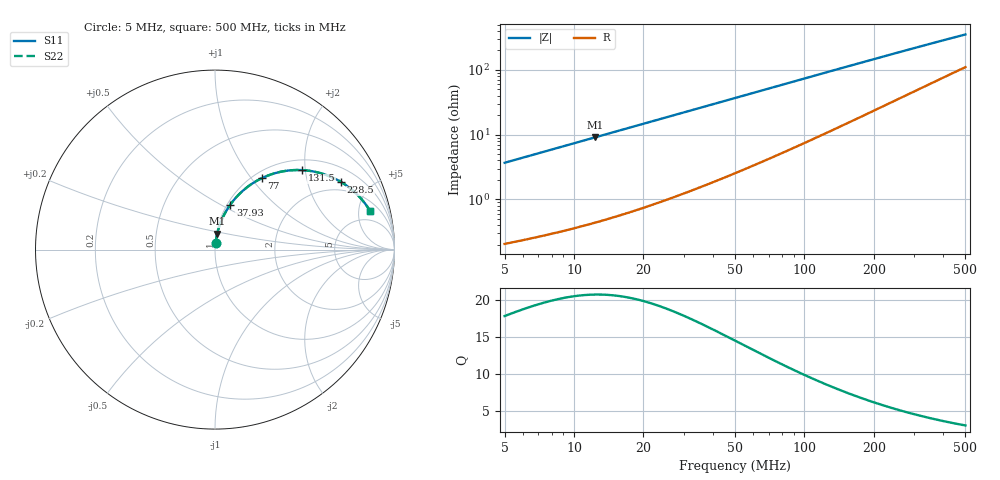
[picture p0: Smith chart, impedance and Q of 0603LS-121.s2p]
# MHz S MA R 50
!Freq  MagS11  AngS11  MagS21  AngS21  MagS12  AngS12  MagS22  AngS22
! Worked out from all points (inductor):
!   801 points, 5 MHz to 500 MHz, reference 50 ohm
!   read as one part in series: L = 117 nH near 5.116 MHz
!   highest Q = 20.7 at 12.34 MHz (marker M1), where L = 117 nH
!   S11 on the Smith chart (normalised r, x): 5 MHz: 1.00, +0.07; 37.93 MHz: 1.03, +0.56; 77 MHz: 1.10, +1.13; 131.5 MHz: 1.23, +1.92; 228.5 MHz: 1.59, +3.27; 500 MHz: 3.20, +6.67
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5  0.0367 84.7  0.9973 -2.1  0.9973 -2.1  0.0367 84.7
6.55345  0.04806 84.3  0.9963 -2.8  0.9963 -2.8  0.04806 84.3
8.202949  0.06011 83.7  0.9952 -3.4  0.9952 -3.4  0.06011 83.7
10.15009  0.07428 83.0  0.9936 -4.3  0.9936 -4.3  0.07428 83.0
12.3444  0.09019 82.1  0.9916 -5.2  0.9916 -5.2  0.09019 82.1
17.04002  0.1239 80.1  0.9862 -7.1  0.9862 -7.1  0.1239 80.1
22.85441  0.1648 77.6  0.9778 -9.5  0.9778 -9.5  0.1648 77.6
29.78311  0.2121 74.6  0.9655 -12.2  0.9655 -12.2  0.2121 74.6
37.92888  0.2653 71.2  0.9482 -15.4  0.9482 -15.4  0.2653 71.2
46.12857  0.3157 67.8  0.9282 -18.4  0.9282 -18.4  0.3157 67.8
55.14041  0.3674 64.4  0.9039 -21.5  0.9039 -21.5  0.3674 64.4
76.99633  0.4759 56.7  0.8394 -28.3  0.8394 -28.3  0.4759 56.7
87.89618  0.5214 53.4  0.8061 -31.3  0.8061 -31.3  0.5214 53.4
108.1359  0.5924 47.8  0.7453 -36.1  0.7453 -36.1  0.5924 47.8
131.5134  0.6562 42.5  0.6799 -40.6  0.6799 -40.6  0.6562 42.5
170.4002  0.7307 35.5  0.5861 -46.3  0.5861 -46.3  0.7307 35.5
197.911  0.7671 31.6  0.5311 -49.2  0.5311 -49.2  0.7671 31.6
228.5441  0.7972 28.2  0.4794 -51.7  0.4794 -51.7  0.7972 28.2
253.4954  0.816 25.8  0.4435 -53.2  0.4435 -53.2  0.816 25.8
336.1012  0.856 20.2  0.3544 -56.3  0.3544 -56.3  0.856 20.2
418.2828  0.8778 16.5  0.2952 -57.6  0.2952 -57.6  0.8778 16.5
500  0.891 14.0  0.2538 -57.8  0.2538 -57.8  0.891 14.0
